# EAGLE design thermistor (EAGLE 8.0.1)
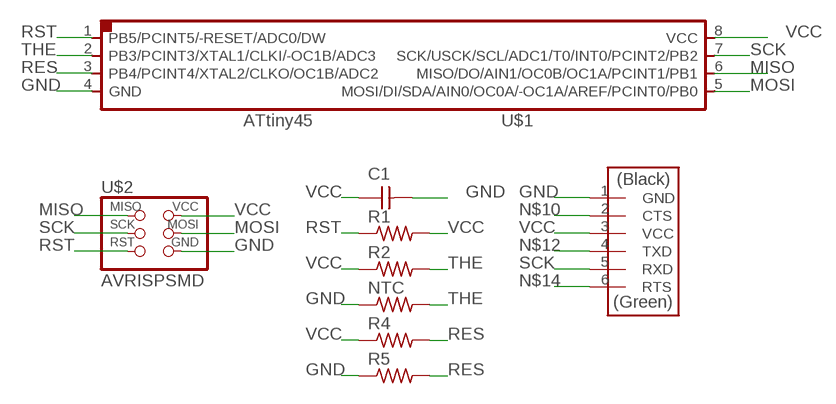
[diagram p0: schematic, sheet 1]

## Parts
C1  CAP-UNPOLARIZEDFAB  [C1206FAB]
NTC  RES-US1206FAB  [R1206FAB]
R1  RES-US1206FAB  [R1206FAB]
R2  RES-US1206FAB  [R1206FAB]
R4  RES-US1206FAB  [R1206FAB]
R5  RES-US1206FAB  [R1206FAB]
U$1  ATTINY45SI  [SOIC8]
U$2  AVRISPSMD  [2X03SMD]
U$3  FTDI-SMD-HEADER  [1X06SMD]

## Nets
GND: C1.2 NTC.1 R5.1 U$1.4(GND) U$2.6(GND) U$3.1(GND)
MISO: U$1.6(MISO/DO/AIN1/OC0B/OC1A/PCINT1/PB1) U$2.1(MISO)
MOSI: U$1.5(MOSI/DI/SDA/AIN0/OC0A/-OC1A/AREF/PCINT0/PB0) U$2.4(MOSI)
N$10: U$3.2(CTS)
N$12: U$3.4(TXD)
N$14: U$3.6(RTS)
RES: R4.2 R5.2 U$1.3(PB4/PCINT4/XTAL2/CLKO/OC1B/ADC2)
RST: R1.1 U$1.1(PB5/PCINT5/-RESET/ADC0/DW) U$2.5(RST)
SCK: U$1.7(SCK/USCK/SCL/ADC1/T0/INT0/PCINT2/PB2) U$2.3(SCK) U$3.5(RXD)
THE: NTC.2 R2.2 U$1.2(PB3/PCINT3/XTAL1/CLKI/-OC1B/ADC3)
VCC: C1.1 R1.2 R2.1 R4.1 U$1.8(VCC) U$2.2(VCC) U$3.3(VCC)

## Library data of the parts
C1 = fab:CAP-UNPOLARIZED
NTC R1 R2 R4 R5 = fab:RES-US: Resistor (US Symbol)
U$1 = fab:ATTINY45
U$2 = fab:AVRISP
U$3 = fab:FTDI-SMD-HEADER

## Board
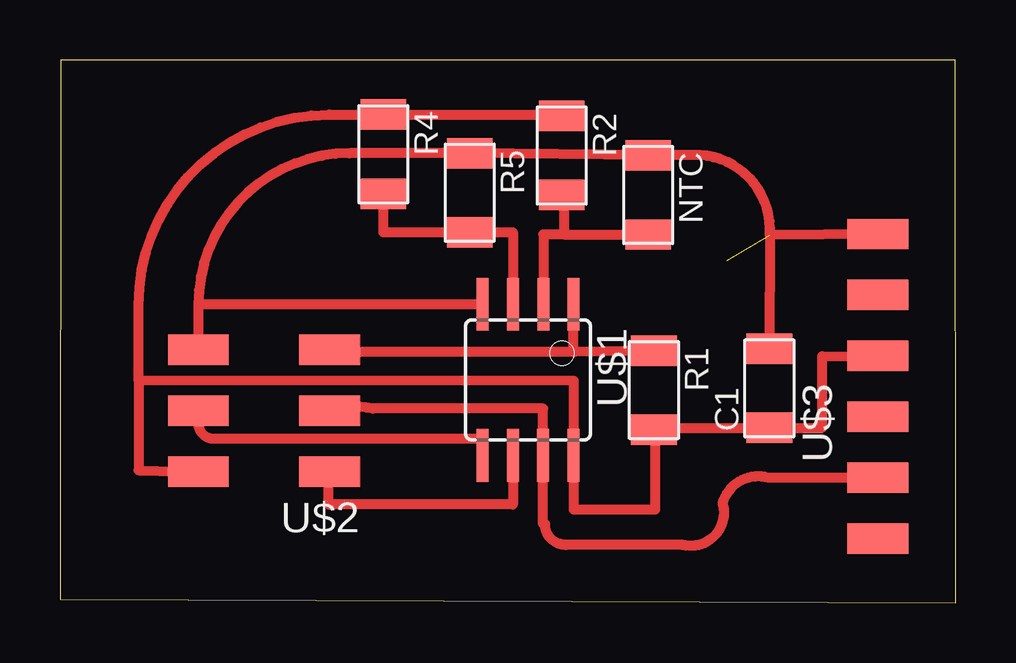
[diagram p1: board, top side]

Size 37.34 x 22.64 mm. Coordinates in mm from the lower left corner, seen from the top.
Outline: 0,0.16 37.34,0 37.32,22.62 0.04,22.64 0,0.16
Copper layers (1*16): Top 0.035mm / dielectric 1.5mm / Bottom 0.035mm
Design rules "default": minimum track width 10mil, minimum drill 24mil, track to track 8mil, track to pad 8mil, pad to pad 8mil, via to via 8mil, smd to smd 8mil, copper to edge 40mil, drill to drill 8mil, minimum pad ring 10mil, minimum via ring 8mil, stop-mask expansion 4mil, vias tented up to drill 0mil, thermal gap 10mil

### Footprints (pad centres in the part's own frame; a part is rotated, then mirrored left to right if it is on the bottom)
C1206FAB = smd 1.27 x 1.905: 1 -1.651,0; 2 1.651,0
R1206FAB = smd 1.27 x 1.905: 1 -1.651,0; 2 1.651,0
SOIC8 = smd 0.5 x 2.2: 1 -1.905,-3.154; 2 -0.645,-3.154; 3 0.625,-3.154; 4 1.895,-3.154; 5 1.905,3.154; 6 0.635,3.154; 7 -0.635,3.154; 8 -1.905,3.154
2X03SMD = smd 2.54 x 1.27: 1 -2.54,2.54; 2 2.92,2.54; 3 -2.54,0; 4 2.92,0; 5 -2.54,-2.54; 6 2.92,-2.54
1X06SMD = smd 2.54 x 1.27: 1 0,6.35; 2 0,3.81; 3 0,1.27; 4 0,-1.27; 5 0,-3.81; 6 0,-6.35

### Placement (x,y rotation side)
C1  29.57,8.95 90 top
NTC  24.52,17.01 270 top
R1  24.76,8.87 270 top
R2  20.92,18.66 270 top
R4  13.48,18.71 270 top
R5  17.08,17.1 270 top
U$1  19.51,9.3 180 top
U$2  8.69,8.01 180 top
U$3  34.1,9.03 0 top

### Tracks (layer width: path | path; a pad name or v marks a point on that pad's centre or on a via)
GND  (1 unrouted)
  Top 0.406: 5.77,12.45 U$1.4 | 5.77,12.45 U$2.6 | U$3.1 29.59,15.34 | 29.59,15.34 C1.2 | 29.59,15.34 arc90 26.69,18.68 NTC.1 R5.1 12.07,18.75 arc90 5.77,12.45
MISO
  Top 0.406: U$1.6 18.88,4.1 11.2,4.1 11.2,5.53 U$2.1
MOSI
  Top 0.406: U$1.5 17.61,6.84 6.42,6.84 arc-90 5.77,7.49 U$2.4
RES
  Top 0.406: U$1.3 18.89,15.45 R5.2 13.48,15.45 R4.2
RST
  Top 0.406: 21.41,10.46 U$1.1 | U$2.5 11.29,10.48 21.48,10.48 21.41,10.46 | R1.1 21.41,10.46
SCK
  Top 0.406: U$2.3 arc-30 13.04,8.1 20.14,8.1 U$1.7 20.14,3.28 20.22,3.28 arc90 21.08,2.42 25.96,2.42 arc121 27.62,4.16 arc-90 29.54,5.22 U$3.5
THE
  Top 0.406: 21.02,15.36 NTC.2 | 21.02,15.36 20.16,15.36 U$1.2 | R2.2 21.02,17.01 21.02,15.36
VCC
  Top 0.406: 3.28,9.28 21.41,9.26 U$1.8 21.41,3.9 24.82,3.9 24.82,7.36 R1.2 24.76,7.3 C1.1 31.78,7.3 31.78,10.28 U$3.3 | 3.28,9.28 3.28,5.53 U$2.2 | 3.28,9.28 3.28,12.42 arc-90 11.22,20.36 R4.1 arc90 R4.1 20.87,20.36 arc-90 R2.1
